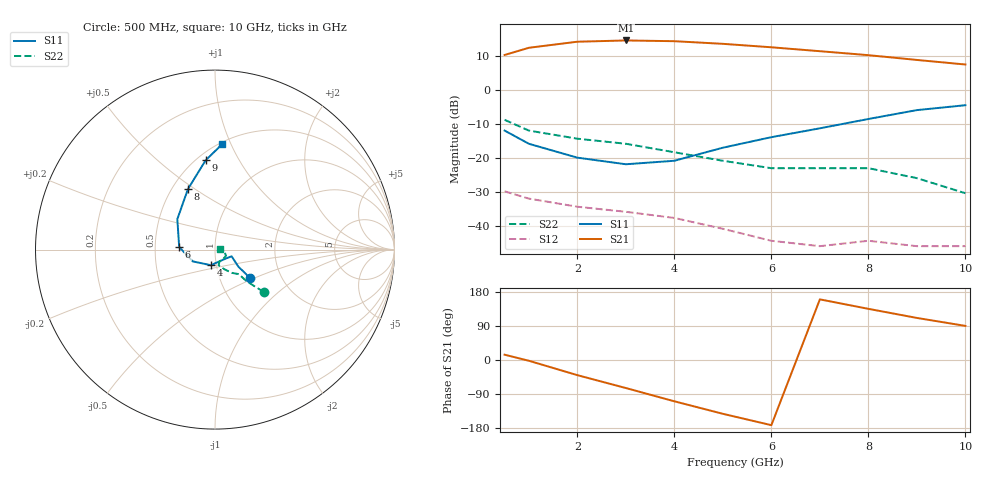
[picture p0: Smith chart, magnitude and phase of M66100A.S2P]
!  MGA-66100 S PARAMETERS
!  Vd=8V  Id=200mA  LAST UPDATED 07-22-92
# ghz s ma r 50
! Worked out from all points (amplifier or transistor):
!   11 points, 500 MHz to 10 GHz, reference 50 ohm
!   highest |S21| = 14.5 dB at 3 GHz (marker M1)
!   |S21| within 3 dB of that: 800.1 MHz to 6.862 GHz (6.061 GHz wide, 158 % of centre)
!   unconditionally stable (mu >= 1): start of sweep to end of sweep
!   at 1 GHz: K = 4.47, MAG = 12.7 dB, |S12| = -32.0 dB
!   at 5 GHz: K = 11.49, MAG = 13.6 dB, |S12| = -40.9 dB
!   at 10 GHz: K = 27.84, MAG = 9.2 dB, |S12| = -46.0 dB
!   S11 on the Smith chart (normalised r, x): 500 MHz: 1.39, -0.47; 4 GHz: 0.94, -0.16; 6 GHz: 0.67, +0.02; 8 GHz: 0.60, +0.47; 9 GHz: 0.55, +0.73; 10 GHz: 0.52, +0.93
0.5  0.25 -39.0  3.23 14.0  0.032 -8.0  0.36 -41.0
1  0.16 -36.0  4.12 -2.0  0.025 -17.0  0.25 -45.0
2  0.1 -22.0  5.06 -40.0  0.019 -14.0  0.19 -46.0
3  0.08 -37.0  5.28 -74.0  0.016 -11.0  0.16 -54.0
4  0.09 -105.0  5.15 -109.0  0.013 -9.0  0.12 -65.0
5  0.14 -152.0  4.71 -142.0  0.009 2.0  0.09 -77.0
6  0.2 176.0  4.19 -172.0  0.006 18.0  0.07 -69.0
7  0.27 141.0  3.67 160.0  0.005 54.0  0.07 -48.0
8  0.37 114.0  3.21 135.0  0.006 67.0  0.07 -28.0
9  0.5 96.0  2.73 111.0  0.005 90.0  0.05 -10.0
10  0.59 86.0  2.34 90.0  0.005 100.0  0.03 7.0
